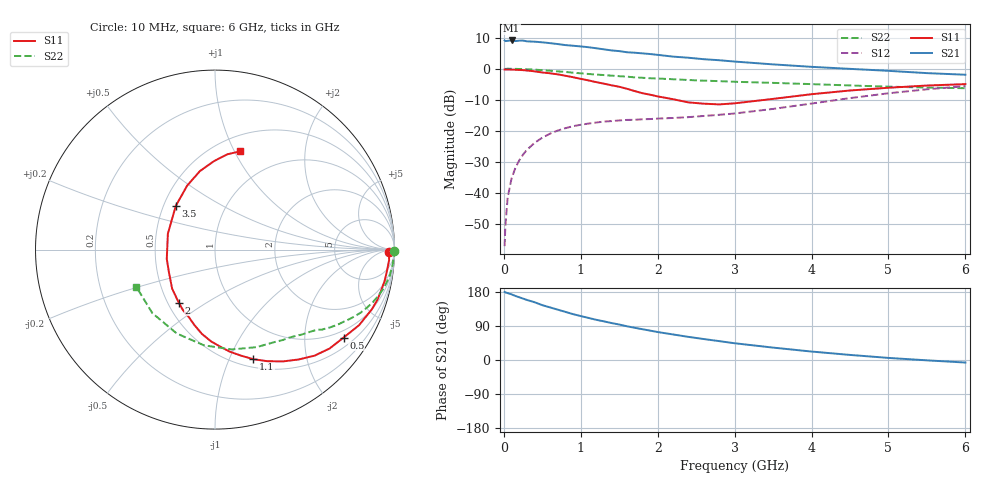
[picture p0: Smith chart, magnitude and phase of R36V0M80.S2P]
! SIEMENS Small Signal Semiconductors
! BFR181
! Si NPN RF Bipolar Junction Transistor in SOT23
! VCE = 6 V  IC = 0.8 mA
! Common Emitter S-Parameters:  May  1996
# GHz  S  MA  R  50
!  f  S11  S21  S12  S22
! GHz  MAG  ANG  MAG  ANG  MAG  ANG  MAG  ANG
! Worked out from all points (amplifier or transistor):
!   36 points, 10 MHz to 6 GHz, reference 50 ohm
!   highest |S21| = 9.1 dB at 100 MHz (marker M1)
!   |S21| within 3 dB of that: start of sweep to 1.342 GHz
!   unconditionally stable (mu >= 1): 2.168 GHz to 3.766 GHz
!   at 250 MHz: K = 0.14, MSG = 18.3 dB, |S12| = -27.6 dB
!   at 1.4 GHz: K = 0.70, MSG = 11.4 dB, |S12| = -16.9 dB
!   at 6 GHz: K = 0.88, MSG = 1.8 dB, |S12| = -5.6 dB
!   S11 on the Smith chart (normalised r, x): 10 MHz: 54, -25; 500 MHz: 0.77, -3.05; 1.1 GHz: 0.59, -1.23; 2 GHz: 0.57, -0.39; 3.5 GHz: 0.58, +0.31; 6 GHz: 0.65, +1.05
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0.01  0.97 -0.8  2.841 179.5  0.0014 88.8  0.9989 -0.4
0.02  0.9693 -1.3  2.773 178.4  0.003 83.1  0.9892 -0.7
0.05  0.9719 -3.5  2.803 176.5  0.0085 87.3  0.9979 -1.7
0.1  0.9657 -7.0  2.842 173.3  0.0171 86.5  0.9948 -3.3
0.15  0.9611 -10.4  2.778 169.0  0.0254 82.2  0.9929 -5.1
0.25  0.9464 -17.4  2.831 162.0  0.0416 77.9  0.9847 -8.3
0.3  0.9349 -20.9  2.748 158.5  0.0496 76.2  0.978 -9.9
0.4  0.9064 -27.7  2.716 152.4  0.0642 71.7  0.9649 -12.9
0.5  0.8679 -34.4  2.653 144.7  0.0778 67.9  0.9455 -15.8
0.7  0.8105 -46.8  2.488 132.9  0.1011 60.2  0.9054 -21.0
0.9  0.7291 -58.7  2.338 121.0  0.1189 53.9  0.8628 -25.5
1.1  0.6468 -70.7  2.213 111.1  0.1311 49.3  0.8216 -29.3
1.4  0.5403 -87.1  1.965 97.5  0.1436 44.0  0.7725 -34.2
1.6  0.4748 -98.9  1.836 89.0  0.15 42.1  0.7446 -36.8
2  0.3581 -124.3  1.667 73.8  0.1576 41.4  0.6945 -41.7
2.2  0.323 -137.7  1.563 67.4  0.1612 41.9  0.6758 -44.5
2.4  0.2869 -153.3  1.499 61.0  0.1662 43.3  0.6572 -47.1
2.8  0.2664 175.1  1.367 49.8  0.1812 46.3  0.6302 -53.0
3.5  0.3268 132.0  1.172 32.7  0.2255 50.6  0.5911 -66.8
4.5  0.4458 100.8  0.993 13.4  0.3364 48.4  0.5371 -96.5
5.5  0.5356 82.6  0.848 -0.9  0.4658 36.2  0.4971 -134.6
6  0.5643 75.8  0.799 -6.7  0.5237 28.1  0.485 -154.6
